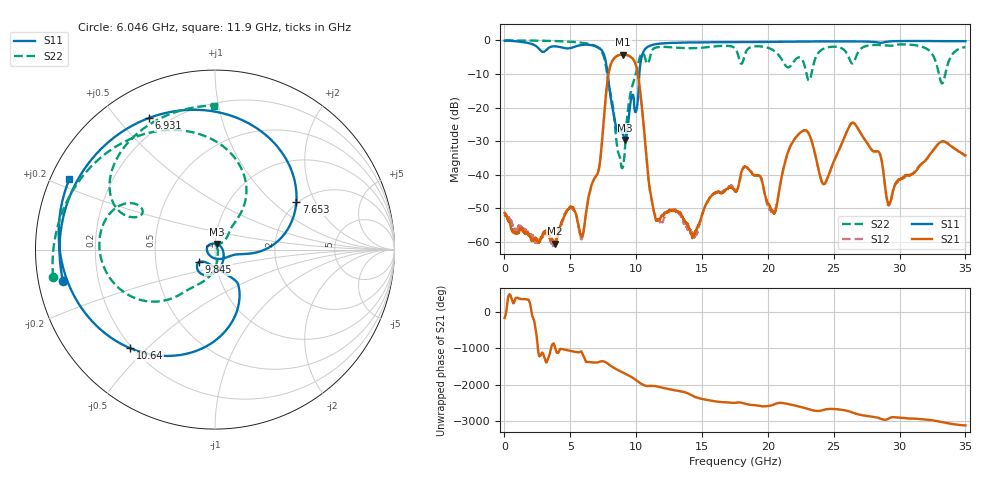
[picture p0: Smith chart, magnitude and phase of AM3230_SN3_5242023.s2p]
!Keysight Technologies,N5245B,MY58422270,A.16.20.02
!Date: Thursday, May 25, 2023 04:43:15
!Correction: S11(C  2-Port  )
!S21(C  2-Port  )
!S12(C  2-Port  )
!S22(C  2-Port  )
!S2P File: Measurements: S11, S21, S12, S22:
# Hz S  dB  R 50
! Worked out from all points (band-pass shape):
!   6401 points, 10 MHz to 35 GHz, reference 50 ohm
!   highest |S21| = -4.18 dB at 9.004 GHz (marker M1); lowest = -60.5 dB at 3.815 GHz (marker M2)
!   |S21| within 3 dB of the highest: 8.066 GHz to 9.97 GHz (1.904 GHz wide, 21.1 % of centre)
!   lowest |S11| = -29.7 dB at 9.162 GHz (marker M3), VSWR 1.07, Z = 50.9 + j3.19 ohm
!   |S11| at or under -10 dB: 7.831 GHz to 10.24 GHz (2.41 GHz wide, 26.7 % of centre)
!   |S22| runs from -38.0 to 0.0 dB; largest |S21 - S12| = 0.0051
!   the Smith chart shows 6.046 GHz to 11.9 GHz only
!   S11 on the Smith chart (normalised r, x): 6.046 GHz: 0.07, -0.10; 6.931 GHz: 0.14, +0.61; 7.653 GHz: 1.96, +1.44; 9.845 GHz: 0.83, -0.12; 10.64 GHz: 0.19, -0.44; 11.9 GHz: 0.05, +0.23
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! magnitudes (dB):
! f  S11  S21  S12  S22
! 10 MHz  -0.1  -51.3  -52.0  -0.1
! 3.815 GHz  -1.7  -60.5  -61.0  -0.2
! 4.952 GHz  -2.3  -49.7  -49.9  -0.4
! 5.843 GHz  -1.3  -58.6  -59.3  -0.7
! 6.046 GHz  -1.3  -55.8  -55.4  -0.8
! 6.931 GHz  -1.7  -40.5  -40.3  -1.7
! 7.653 GHz  -5.6  -18.3  -18.3  -6.6
! 9.004 GHz  -28.0  -4.2  -4.2  -37.4
! 9.162 GHz  -29.7  -4.2  -4.2  -31.3
! 9.845 GHz  -18.9  -6.0  -6.0  -11.7
! 10.64 GHz  -2.8  -28.1  -28.1  -4.7
! 11.68 GHz  -1.0  -53.2  -53.2  -2.0
! 11.9 GHz  -0.9  -52.4  -54.1  -1.9
! 17.5 GHz  -0.5  -44.9  -44.5  -2.4
! 20.47 GHz  -0.4  -51.6  -51.0  -3.1
! 21.82 GHz  -0.3  -30.7  -30.6  -7.1
! 23.34 GHz  -0.3  -30.1  -30.1  -9.4
! 24.27 GHz  -0.3  -42.7  -42.9  -2.4
! 26.58 GHz  -0.3  -24.7  -24.7  -6.1
! 29.17 GHz  -0.3  -49.0  -49.0  -1.6
! 33.23 GHz  -0.2  -30.0  -30.1  -12.8
! 35 GHz  -0.2  -34.2  -34.4  -2.0
